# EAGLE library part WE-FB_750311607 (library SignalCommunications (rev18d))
WE-FB Flyback Transformer suitable for LT3573/ LT3574/ LT3575/ LT3748 Characteristics easy design in solution less external components needed small board space low cost no optocoupler needed! long term reliability voltage control no aging same external parts for different output voltages easy design of custom power supply due to standard circuit and change of transformers and two components for feedback loop Isolation voltage up to 2.5 kV Applications Isolated power design Sensor interfaces Isolated telecom converters Power over Ethernet Details see: http://katalog.we-online.de/en/pbs/WE-FB_Linear? Updated 2015-04-03 2015 (C) Wurth Elektronik
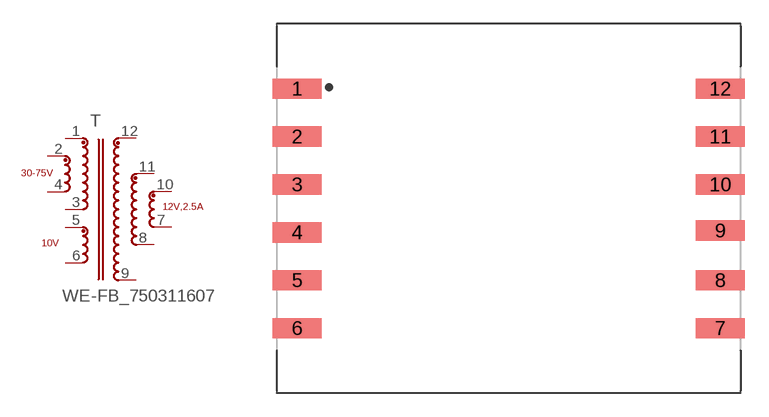
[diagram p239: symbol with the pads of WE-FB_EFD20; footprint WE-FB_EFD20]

Designator prefix T

## WE-FB_750311607  [WE-FB_EFD20]
1  2  pas
2  1  pas
3  11  pas
4  12  pas
5  10  pas
6  9  pas
7  6  pas
8  7  pas
9  8  pas
10  5  pas
11  4  pas
12  3  pas

## Footprint WE-FB_EFD20 (pad centres in mm)
smd 3.05 x 1.27: 1 -13.26,7.5; 2 -13.26,4.5; 3 -13.26,1.5; 4 -13.26,-1.5; 5 -13.26,-4.5; 6 -13.26,-7.5; 7 13.26,-7.5; 8 13.26,-4.5; 9 13.26,-1.39; 10 13.26,1.5; 11 13.26,4.5; 12 13.26,7.5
